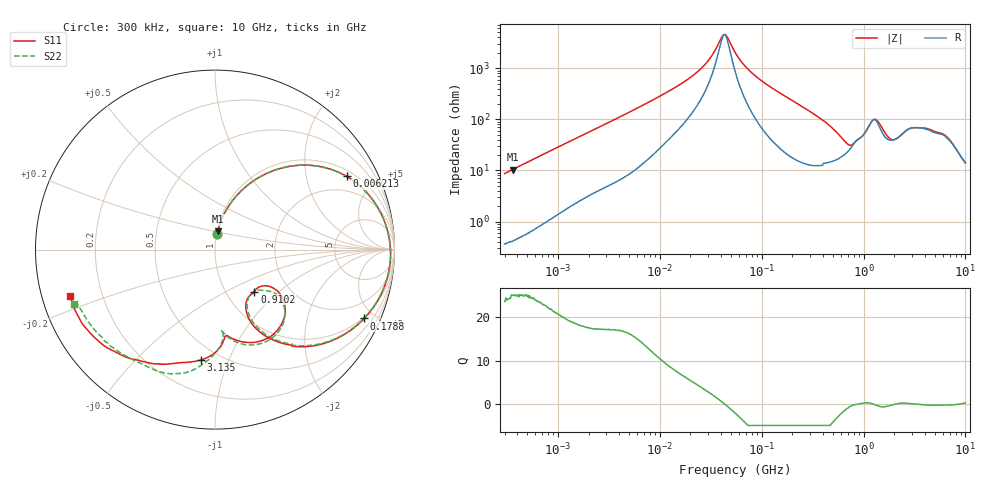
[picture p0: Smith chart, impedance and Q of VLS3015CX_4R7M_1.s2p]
! S-Parameter Data Generated by TDK Corporation
! Copyright(C) 2019 TDK Corporation.
! All Rights Reserved.
! TDK P/N: VLS3015CX-4R7M-1 (Inductor)
! Property: L=4.7uH at 1MHz
! Size(LxWxT): 3x3x1.5mm
! Model Type: s2p (Touchstone File Format Version 1.0)
! Frequency: DC=Yes Start=0.3MHz Stop=10000MHz 802points Log-sweep
! Model Generated on Sep. 23, 2019
! Port Assignments:
!  1 ---@@@--- 2
! Applicable Conditions:
!  Temperature = 25 degC
!  DC Bias Current = 0 A
!  Small Signal Operation
! Terms and conditions regarding TDK Simulation Models
! (1)This simulation model is being provided solely for informational purposes. Please refer to the specifications of the products in terms of detailed characteristics of such products.
! (2)In no event shall TDK Corporation of any of its subsidiaries be liable for any loss or damage arising, directly or indirectly,
!  From any information contained in this simulation model, including, but not limited to loss or damages arising from any inaccuracies, omissions or errors in connection with such information.
! (3)Any and all copyrights on this simulation model are owned by TDK Corporation.
!  Duplication or redistribution of this simulation model without prior written permission from TDK Corporation is prohibited.
! (4)This simulation model is subject to any modification or change without any prior notice.
! (5)Neither TDK Corporation nor any of its subsidiaries shall make any warranty, express or implied,
!  Including but not limited to the correctness, implied warranties of merchantability and fitness for a particular purpose with respect to this simulation models.
! (6)The use of this simulation model shall be deemed to have consented to the terms and conditions hereof.
# Hz S MA R 50
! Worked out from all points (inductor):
!   801 points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, 300 kHz to 10 GHz, reference 50 ohm
!   read as one part in series: L = 4.6 uH near 318.3 kHz
!   highest Q = 25.1 at 359.6 kHz (marker M1), where L = 4.6 uH
!   self-resonance near 43.13 MHz
!   S11 on the Smith chart (normalised r, x): 300 kHz: 1.01, +0.17; 6.213 MHz: 1.24, +3.43; 178.8 MHz: 0.92, -4.37; 910.2 MHz: 1.35, -0.70; 3.135 GHz: 0.40, -0.80; 10 GHz: 0.09, -0.16
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300000  0.08617 82.5  0.9926 -5.0  0.9926 -4.9  0.08593 82.6
359595  0.1029 81.8  0.9906 -5.9  0.9906 -5.9  0.1027 81.7
1713600  0.424 61.7  0.8824 -25.1  0.8825 -25.1  0.424 61.7
6213199  0.839 29.1  0.4902 -57.0  0.4903 -57.0  0.839 29.1
9671944  0.9118 19.2  0.3346 -65.5  0.3346 -65.5  0.9118 19.2
2.473055e7  0.9698 5.1  0.1038 -70.9  0.1038 -70.9  0.9698 5.1
4.259986e7  0.9785 -1.1  0.0216 -6.9  0.0216 -6.9  0.9785 -1.0
5.477226e7  0.9786 -4.0  0.04762 60.6  0.04763 60.6  0.9785 -4.0
8.505279e7  0.9716 -10.0  0.1325 71.5  0.1325 71.5  0.9715 -9.8
1.788252e8  0.9159 -24.8  0.3377 61.0  0.3378 61.0  0.9158 -24.5
3.126428e8  0.786 -42.4  0.5524 42.8  0.5524 42.8  0.7861 -41.9
6.15965e8  0.4379 -63.8  0.7622 7.5  0.7623 7.5  0.4371 -62.6
7.612374e8  0.3272 -56.3  0.7469 -7.1  0.747 -7.1  0.3213 -53.1
9.101824e8  0.3208 -46.7  0.6816 -16.1  0.6818 -16.1  0.3528 -40.4
1.10164e9  0.3875 -33.4  0.5794 -27.0  0.5792 -27.0  0.4433 -36.4
1.276148e9  0.5337 -43.2  0.4644 -22.4  0.4641 -22.4  0.5658 -48.5
1.767019e9  0.5141 -77.5  0.6099 -23.9  0.6097 -23.9  0.498 -81.1
2.294622e9  0.4878 -83.5  0.5731 -44.8  0.573 -44.7  0.4578 -84.8
3.135132e9  0.6212 -97.4  0.4214 -57.0  0.4219 -57.0  0.6094 -92.8
4.34106e9  0.7024 -114.4  0.3446 -62.7  0.3452 -62.7  0.733 -109.3
6.333834e9  0.7752 -129.2  0.2866 -76.4  0.2865 -76.6  0.776 -131.0
1e10  0.8466 -162.2  0.2226 -97.0  0.2215 -96.9  0.8416 -158.8
